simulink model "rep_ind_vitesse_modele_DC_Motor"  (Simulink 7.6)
settings: Solver=ode15s  StartTime=0.0  StopTime=100  RelTol=1e-3
PreLoadFcn:
  | close all
  | clc
  | clear all
InitFcn:
  | % échelon
  | echelon=12;
  | 
  | % caractéristiques électriques du moteur
  | R=3.9;         % résistance d'induit (ohm)
  | L= 1.2e-05; % inductance d'induit (H)
  | E=7.2e-05;  % fcem  (V/rpm)
  | 
  | % caractéristiques mécaniques du moteur
  | J1=0.01;      % inertie du rotor (g*cm^2)
  | f1=1e-08       % amortissement (N*m/(rad/s))
  | 
  | % inertie rajoutée sur l'arbre moteur
  | Jext=10;      % inertie externe (g*cm^2)
StopFcn:
  | close all, clc
  | load rep_ind_vit.mat
  | plot(x(1,:),x(2,:), x(1,:),x(4,:),'*')
  | grid
  | title('Réponse indicielle de vitesse DC Motor et son modèle')
  | xlabel('temps')
libraries: fl_lib x7, nesl_utility x3, elec_lib x1

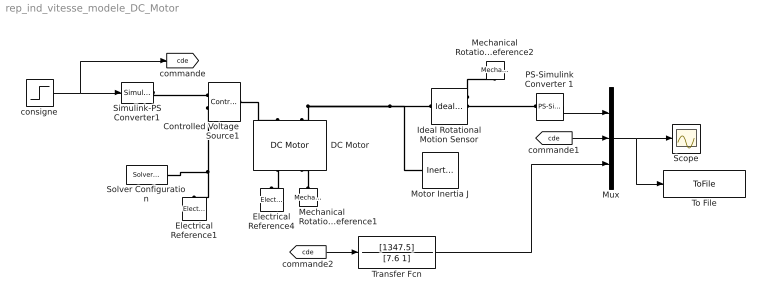
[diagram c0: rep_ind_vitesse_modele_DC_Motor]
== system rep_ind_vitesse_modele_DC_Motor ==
  Controlled Voltage Source1 : fl_lib/Electrical/Electrical Sources/Controlled Voltage Source  DialogController=NetworkEngine.DynNeDlgSource  SystemSampleTime=-1  i_Log=off  v_Log=off  LocalVarNames=|current|voltage|power  LocalVarDescs=|Current (A)|Voltage (V)|Power (W)  LocalVarLogging=[0 0 0]
  DC Motor : elec_lib/Actuators & Drivers/Rotational Actuators/DC Motor  DialogController=NetworkEngine.DynNeDlgSource  SystemSampleTime=-1  parameterization=1  Ra=R Ohm  La=L H  emf_or_torque=1  Kv=E V/rpm  Ki=6.876e-04 N*m/A  T_stall=2.4e-04 N*m  w_max=1.91e+04 rpm  w_rated=1.5e+04 rpm  P_rated=0.08 W  V_rated=1.5 V  J=J1 g*cm^2  lam=f1 N*m/(rad/s)  speed0=0 rpm  current_Log=off  voltage_Log=off  power_Log=off  i2r_Log=off  torque_Log=off  speed_Log=off  LocalVarNames=|current|voltage|power|i2r|torque|speed  LocalVarDescs=|Current (A)|Voltage (V)|Power (W)|Electrical losses (W)|Torque (Nm)|Angular speed (rad/s)  LocalVarLogging=[0 0 0 0 0 0]
  Electrical Reference1 : fl_lib/Electrical/Electrical Elements/Electrical Reference  DialogController=NetworkEngine.DynNeDlgSource  SystemSampleTime=-1  i_Log=off  LocalVarNames=|i  LocalVarDescs=|i  LocalVarLogging=[]
  Electrical Reference4 : fl_lib/Electrical/Electrical Elements/Electrical Reference  DialogController=NetworkEngine.DynNeDlgSource  SystemSampleTime=-1  i_Log=off  LocalVarNames=|i  LocalVarDescs=|i  LocalVarLogging=[]
  Ideal Rotational Motion Sensor : fl_lib/Mechanical/Mechanical Sensors/Ideal Rotational Motion Sensor  DialogController=NetworkEngine.DynNeDlgSource  SystemSampleTime=-1  offset=0 rad  w_Log=off  t_Log=off  phi_Log=off  LocalVarNames=|w|t|phi  LocalVarDescs=|w|t|phi  LocalVarLogging=[0 0 0]
  Mechanical Rotational Reference1 : fl_lib/Mechanical/Rotational Elements/Mechanical Rotational Reference  DialogController=NetworkEngine.DynNeDlgSource  SystemSampleTime=-1  t_Log=off  LocalVarNames=|t  LocalVarDescs=|t  LocalVarLogging=[]
  Mechanical Rotational Reference2 : fl_lib/Mechanical/Rotational Elements/Mechanical Rotational Reference  DialogController=NetworkEngine.DynNeDlgSource  SystemSampleTime=-1  t_Log=off  LocalVarNames=|t  LocalVarDescs=|t  LocalVarLogging=[]
  Motor Inertia J : fl_lib/Mechanical/Rotational Elements/Inertia  DialogController=NetworkEngine.DynNeDlgSource  SystemSampleTime=-1  inertia=Jext g*cm^2  initial_velocity=0 rad/s  t_Log=off  LocalVarNames=|torque|velocity  LocalVarDescs=|Inertia torque (N*m)|Inertia absolute velocity (rad/s)  LocalVarLogging=[0 0]
  Mux : Mux  Inputs=3
  PS-Simulink Converter 1 : nesl_utility/PS-Simulink Converter  DialogController=NetworkEngine.DynNeUtilDlgSource  SystemSampleTime=-1  PhysicalDomain=network_engine_domain  LeftPortType=input  RightPortType=output  SubClassName=ps_output  Unit=1  AffineConversion=off
  Scope : Scope
  Simulink-PS Converter1 : nesl_utility/Simulink-PS Converter  DialogController=NetworkEngine.DynNeUtilDlgSource  SystemSampleTime=-1  PhysicalDomain=network_engine_domain  LeftPortType=input  RightPortType=output  SubClassName=ps_input  Unit=1  AffineConversion=off  InputFilterTimeConstant=.001  UdotUserProvided=0
  Solver Configuration : nesl_utility/Solver Configuration  DialogController=NetworkEngine.DynNeUtilDlgSource  SystemSampleTime=-1  PhysicalDomain=network_engine_domain  LeftPortType=input  RightPortType=generic  SubClassName=solver  Accelerate=off  Profile=off  ResidualTolerance=1e-9  MaxNonlinIter=12  MaxModeIter=2  DoFixedCost=off  UseLocalSampling=off  DoDC=off  LinearAlgebra=Full  LocalSolverSampleTime=.001  LocalSolverChoice=NE_BACKWARD_EULER_ADVANCER  UseLocalSolver=off
  To File : ToFile  Filename=rep_ind_vit.mat  MatrixName=x
  Transfer Fcn : TransferFcn  Numerator=[1347.5]  Denominator=[7.6 1]
  consigne : Step  Time=10  After=echelon  SampleTime=0
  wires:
  PS-Simulink Converter 1/1 -> Mux/1
  Mux/1 -> To File/1, Scope/1
  consigne/1 -> Simulink-PS Converter1/1, [cde]
  [cde] -> Mux/2
  Transfer Fcn/1 -> Mux/3
  [cde] -> Transfer Fcn/1
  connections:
  Ideal Rotational Motion Sensor/RConn1 -- Mechanical Rotational Reference2/LConn1
  Ideal Rotational Motion Sensor/RConn2 -- PS-Simulink Converter 1/LConn1
  Simulink-PS Converter1/RConn1 -- Controlled Voltage Source1/RConn1
  Mechanical Rotational Reference1/LConn1 -- DC Motor/RConn2
  DC Motor/LConn2 -- Motor Inertia J/LConn1 -- Ideal Rotational Motion Sensor/LConn1
  DC Motor/RConn1 -- Electrical Reference4/LConn1
  Controlled Voltage Source1/LConn1 -- DC Motor/LConn1
  Controlled Voltage Source1/RConn2 -- Electrical Reference1/LConn1 -- Solver Configuration/RConn1
